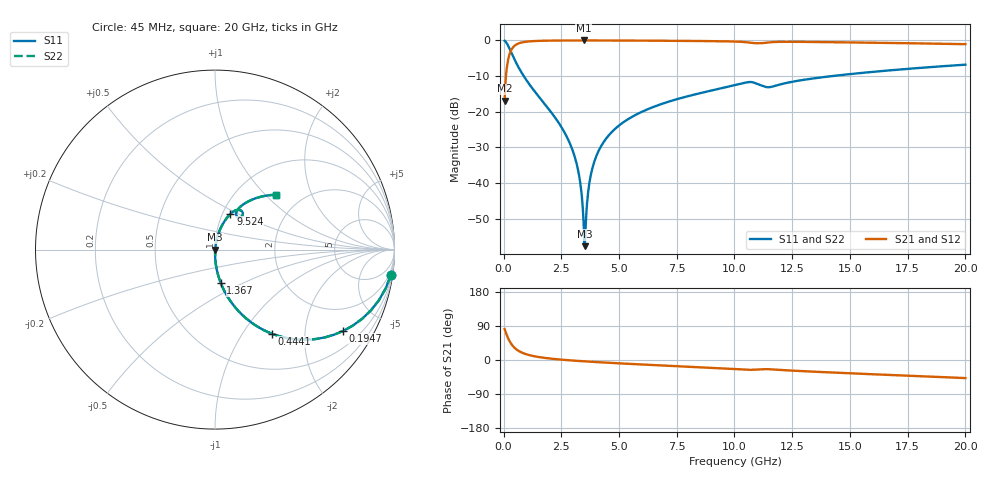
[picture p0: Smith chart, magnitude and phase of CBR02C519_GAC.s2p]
! S-parameter model data by Modelithics Inc.  support@modelithics.com 813-866-6335  Tampa FL USA
! S-Parameter data specifications:
! Substrate: 20-mil Rogers 4350B, substrate thickness, H=0.508mm, Dielectric constant, Er=3.75
! PCB Mounting Pad Footprint: Pad width, PadW=0.32mm , Pad length, PadL=0.37mm , Pad gap, PadG (edge-to-edge)=0.19mm , Reference planes=0.93mm apart
#  GHz  S  MA  R 50
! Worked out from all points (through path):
!   801 points, 45 MHz to 20 GHz, reference 50 ohm
!   highest |S21| = -0.01 dB at 3.462 GHz (marker M1); lowest = -16.9 dB at 45 MHz (marker M2)
!   group delay of S21, straight-line fit = 8.95 ps
!   lowest |S11| = -57.7 dB at 3.512 GHz (marker M3), VSWR 1.00, Z = 50.1 - j0.0162 ohm
!   |S11| at or under -10 dB: 873.2 MHz to 14.22 GHz (13.35 GHz wide, 177 % of centre)
!   |S22| runs from -57.7 to -0.1 dB; largest |S21 - S12| = 0
!   S11 on the Smith chart (normalised r, x): 45 MHz: 1, -14; 194.7 MHz: 0.99, -3.16; 444.1 MHz: 0.99, -1.37; 1.367 GHz: 0.99, -0.38; 9.524 GHz: 1.09, +0.45; 20 GHz: 1.50, +1.16
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0.045  0.9896 -8.3  0.1435 81.7  0.1435 81.7  0.9896 -8.3
0.194662  0.8463 -32.4  0.5323 57.6  0.5323 57.6  0.8463 -32.4
0.4441  0.5664 -55.9  0.8234 34.0  0.8234 34.0  0.5664 -55.9
0.768369  0.3588 -69.6  0.9325 20.2  0.9325 20.2  0.3588 -69.6
1.367019  0.1892 -80.2  0.9809 9.5  0.9809 9.5  0.1892 -80.2
2.863644  0.03649 -88.9  0.998 -0.8  0.998 -0.8  0.03649 -88.9
3.212856  0.01595 -87.8  0.9985 -2.4  0.9985 -2.4  0.01595 -87.8
3.387462  0.006623 -81.9  0.9986 -3.1  0.9986 -3.1  0.006623 -81.9
3.462294  0.002923 -67.0  0.9986 -3.4  0.9986 -3.4  0.002923 -67.0
3.512181  0.001306 -7.1  0.9986 -3.6  0.9986 -3.6  0.001306 -7.1
3.587013  0.00389 66.4  0.9986 -3.9  0.9986 -3.9  0.00389 66.4
3.711731  0.009828 77.9  0.9986 -4.4  0.9986 -4.4  0.009828 77.9
3.83645  0.01569 80.3  0.9985 -4.8  0.9985 -4.8  0.01569 80.3
4.310381  0.03662 81.3  0.9979 -6.5  0.9979 -6.5  0.03662 81.3
5.2333  0.07292 79.3  0.9958 -9.5  0.9958 -9.5  0.07292 79.3
6.704981  0.124 75.2  0.9905 -14.0  0.9905 -14.0  0.124 75.2
9.523625  0.2166 66.6  0.9719 -22.3  0.9719 -22.3  0.2166 66.6
10.0225  0.2361 64.2  0.9637 -23.9  0.9637 -23.9  0.2361 64.2
11.51913  0.2212 56.2  0.9397 -24.4  0.9397 -24.4  0.2212 56.2
13.36496  0.2917 58.4  0.9513 -30.6  0.9513 -30.6  0.2917 58.4
16.68248  0.3795 50.1  0.9218 -39.4  0.9218 -39.4  0.3795 50.1
20  0.4572 41.9  0.886 -47.7  0.886 -47.7  0.4572 41.9
